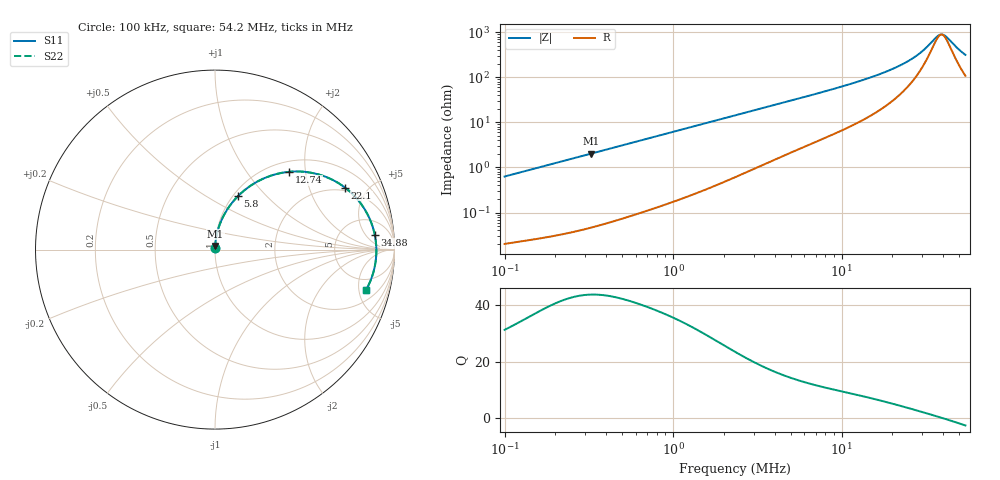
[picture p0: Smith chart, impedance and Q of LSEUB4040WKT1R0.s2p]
! LSEUB4040WKT1R0  S-PARAMETER MODEL  ( Standard Model )
! Model Generated by TAIYO YUDEN Corporation (http://www.ty-top.com)
! Version 1.0
! TAIYO YUDEN Control No. 20230502
! Copyright(c) 2023 TAIYO YUDEN CO.,LTD. All Rights Reserved.
! Product Description (link to TY-COMPAS)
! https://ds.yuden.co.jp/TYCOMPAS/or/detail?pn=LSEUB4040WKT1R0M&u=M
! Products Name : Inductors
! Characteristics :
!  Inductance : 1.0 [uH] , SRF(min) : - [Hz] , DC Resistance(max) : 0.0105 [Ohm]
!  Rated Current : Saturation  10000 [mA] , Temp Rise  7700 [mA] (40 [degC])
!  Case Size : 4.0 x 4.0 / 0.157 x 0.157 [mm/inch] , Thickness : 2.0 / 0.079 [mm/inch]
!  (Conditions: Temperature = 25 [degC] , DC Bias Current = 0 [A])
! External Node Assignments :
!  1  o---GGG---o  2
! GND o---------o GND
! Frequency Range : 0.1MHz  -  54.20166MHz  [ 402 STEP ]
# MHz S RI R 50
! Freq[MHz].  S11 Real  S11 Imag  S21 Real  S21 Imag  S12 Real  S12 Imag  S22 Real  S22 Imag
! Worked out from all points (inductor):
!   401 points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, 100 kHz to 54.2 MHz, reference 50 ohm
!   read as one part in series: L = 997 nH near 103.2 kHz
!   highest Q = 43.8 at 325.6 kHz (marker M1), where L = 988 nH
!   self-resonance near 39.09 MHz
!   S11 on the Smith chart (normalised r, x): 100 kHz: 1.00, +0.01; 5.8 MHz: 1.05, +0.70; 12.74 MHz: 1.20, +1.63; 22.1 MHz: 1.82, +3.53; 34.88 MHz: 11, +9; 54.2 MHz: 3.16, -5.90
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0.1  0.00024 0.00628  0.9998 -0.00628  0.9998 -0.00628  0.00024 0.00628
0.287043  0.000727 0.0178  0.9993 -0.0178  0.9993 -0.0178  0.000727 0.0178
0.325557  0.000869 0.0202  0.9991 -0.0202  0.9991 -0.0202  0.000869 0.0202
0.823937  0.00389 0.0504  0.9961 -0.0504  0.9961 -0.0504  0.00389 0.0504
2.328125  0.0254 0.1375  0.9746 -0.1375  0.9746 -0.1375  0.0254 0.1375
3.852364  0.0635 0.2159  0.9365 -0.2159  0.9365 -0.2159  0.0635 0.2159
5.800135  0.1283 0.298  0.8717 -0.298  0.8717 -0.298  0.1283 0.298
6.682722  0.1617 0.3285  0.8383 -0.3285  0.8383 -0.3285  0.1617 0.3285
9.300131  0.2684 0.3951  0.7316 -0.3951  0.7316 -0.3951  0.2684 0.3951
12.74059  0.4128 0.4334  0.5872 -0.4334  0.5872 -0.4334  0.4128 0.4334
15.88108  0.5351 0.4284  0.4649 -0.4284  0.4649 -0.4284  0.5351 0.4284
19.18229  0.6451 0.3934  0.3549 -0.3934  0.3549 -0.3934  0.6451 0.3934
22.1012  0.7241 0.3458  0.2759 -0.3458  0.2759 -0.3458  0.7241 0.3458
25.46426  0.7938 0.2799  0.2062 -0.2799  0.2062 -0.2799  0.7938 0.2799
28.42996  0.8383 0.2174  0.1617 -0.2174  0.1617 -0.2174  0.8383 0.2174
31.24543  0.8677 0.1573  0.1323 -0.1573  0.1323 -0.1573  0.8677 0.1573
34.88444  0.8902 0.0817  0.1098 -0.0817  0.1098 -0.0817  0.8902 0.0817
37.74043  0.8979 0.0253  0.1021 -0.0253  0.1021 -0.0253  0.8979 0.0253
40.19268  0.8988 -0.0203  0.1012 0.0203  0.1012 0.0203  0.8988 -0.0203
42.13588  0.8964 -0.0545  0.1036 0.0545  0.1036 0.0545  0.8964 -0.0545
50.09997  0.8653 -0.1757  0.1347 0.1757  0.1347 0.1757  0.8653 -0.1757
54.20166  0.8404 -0.2266  0.1596 0.2266  0.1596 0.2266  0.8404 -0.2266
